(* Logix 5000 AddOnInstructionDefinition export AMCI_NXFE2_Absolute_Move; software revision 20.03 *)

ADD_ON_INSTRUCTION AMCI_NXFE2_Absolute_Move   (* revision 1.0, vendor AMCI, ExecuteEnableInFalse *)
VAR_INPUT
   Axis_Status_Bits : INT; {required}
   _0_normal_1_S_curve_acceleration : BOOL;
   _0_triangular_1_trapezoidal_S_curve : BOOL;
   Target_Position : DINT; {required}
   Programmed_Speed : DINT; {required}
   Acceleration : INT; {required}
   Deceleration : INT; {required}
END_VAR
VAR_IN_OUT
   NXFE2_output_data : _000A:NXFE2_0986AEB4:O:0; {required}
END_VAR
VAR_OUTPUT
   EN : BOOL; {access Read Only, visible}
   ER : BOOL; {access Read Only, visible}
END_VAR
VAR
   command_data_block : INT[10];
        [0]   // Command Bits MSW
        [1]   // Command Bits LSW
        [2]   // Upper Target Position
        [3]   // Lower Target Position
        [4]   // Upper Programmed Speed
        [5]   // Lower Programmed Speed
END_VAR

ROUTINE EnableInFalse   (* ladder *)
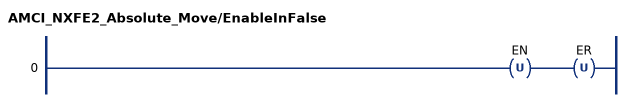
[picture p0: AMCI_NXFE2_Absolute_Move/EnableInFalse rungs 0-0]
   0: OTU(EN)OTU(ER);
END_ROUTINE

ROUTINE Logic   (* ladder *)
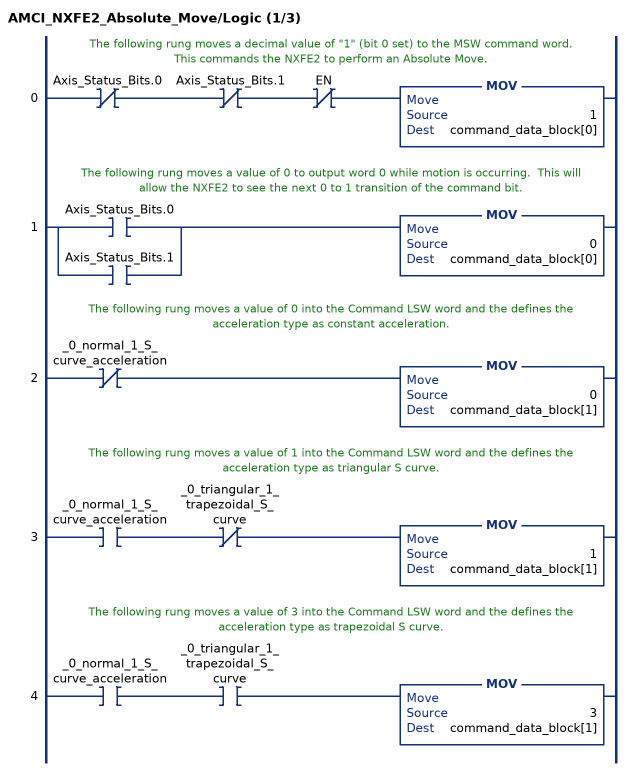
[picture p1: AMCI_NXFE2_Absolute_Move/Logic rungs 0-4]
   // The following rung moves a decimal value of "1" (bit 0 set) to the MSW command word.  This commands the NXFE2 to perform an Absolute Move.
   0: XIO(Axis_Status_Bits.0)XIO(Axis_Status_Bits.1)XIO(EN)MOV(1,command_data_block[0]);
   // The following rung moves a value of 0 to output word 0 while motion is occurring.  This will allow the NXFE2 to see the next 0 to 1 transition of the command bit.
   1: [XIC(Axis_Status_Bits.0) ,XIC(Axis_Status_Bits.1) ]MOV(0,command_data_block[0]);
   // The following rung moves a value of 0 into the Command LSW word and the defines the acceleration type as constant acceleration.
   2: XIO(_0_normal_1_S_curve_acceleration)MOV(0,command_data_block[1]);
   // The following rung moves a value of 1 into the Command LSW word and the defines the acceleration type as triangular S curve.
   3: XIC(_0_normal_1_S_curve_acceleration)XIO(_0_triangular_1_trapezoidal_S_curve)MOV(1,command_data_block[1]);
   // The following rung moves a value of 3 into the Command LSW word and the defines the acceleration type as trapezoidal S curve.
   4: XIC(_0_normal_1_S_curve_acceleration)XIC(_0_triangular_1_trapezoidal_S_curve)MOV(3,command_data_block[1]);
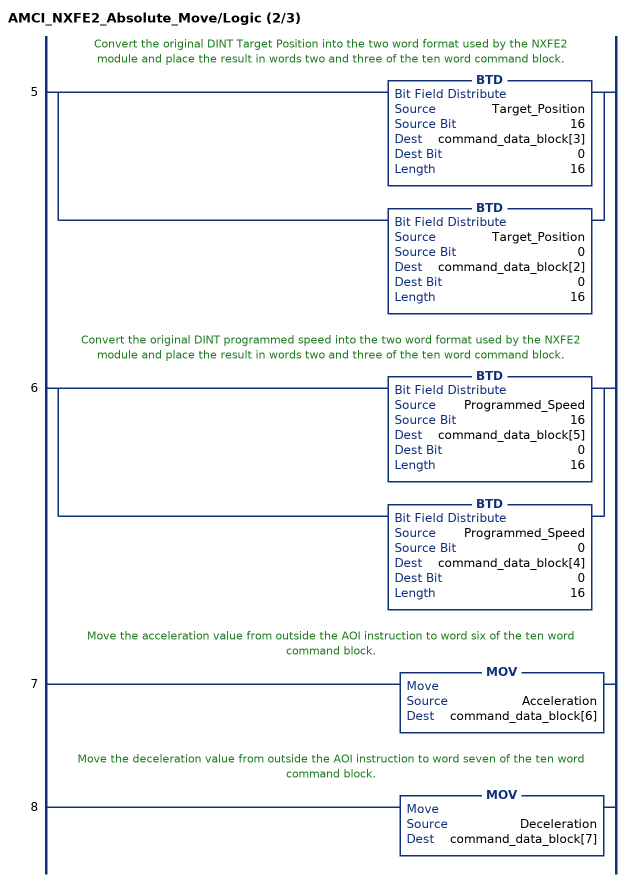
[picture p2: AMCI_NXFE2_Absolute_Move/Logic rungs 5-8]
   // Convert the original DINT Target Position into the two word format used by the NXFE2 module and place the result in words two and three of the ten word command block.
   5: [BTD(Target_Position,16,command_data_block[3],0,16) ,BTD(Target_Position,0,command_data_block[2],0,16) ];
   // Convert the original DINT programmed speed into the two word format used by the NXFE2 module and place the result in words two and three of the ten word command block.
   6: [BTD(Programmed_Speed,16,command_data_block[5],0,16) ,BTD(Programmed_Speed,0,command_data_block[4],0,16) ];
   // Move the acceleration value from outside the AOI instruction to word six of the ten word command block.
   7: MOV(Acceleration,command_data_block[6]);
   // Move the deceleration value from outside the AOI instruction to word seven of the ten word command block.
   8: MOV(Deceleration,command_data_block[7]);
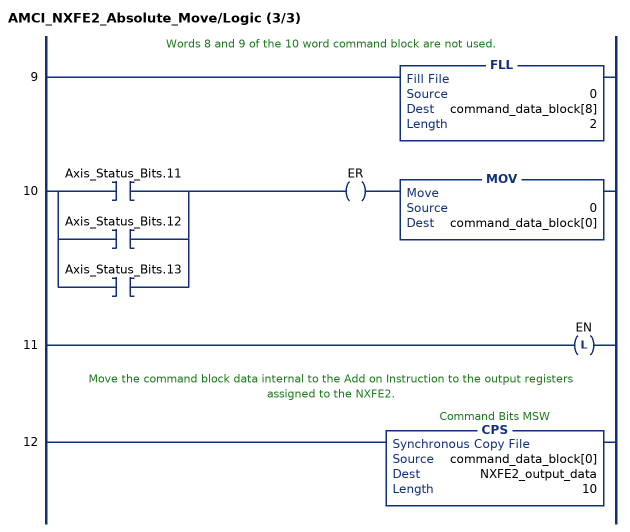
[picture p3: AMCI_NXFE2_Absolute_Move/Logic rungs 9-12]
   // Words 8 and 9 of the 10 word command block are not used.
   9: FLL(0,command_data_block[8],2);
   10: [XIC(Axis_Status_Bits.11) ,XIC(Axis_Status_Bits.12) ,XIC(Axis_Status_Bits.13) ]OTE(ER)MOV(0,command_data_block[0]);
   11: OTL(EN);
   // Move the command block data internal to the Add on Instruction to the output registers assigned to the NXFE2.
   12: CPS(command_data_block[0],NXFE2_output_data,10);
END_ROUTINE
END_ADD_ON_INSTRUCTION
